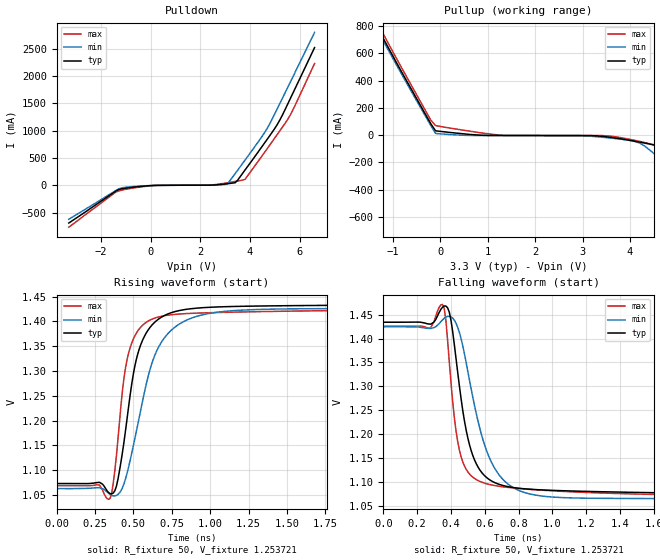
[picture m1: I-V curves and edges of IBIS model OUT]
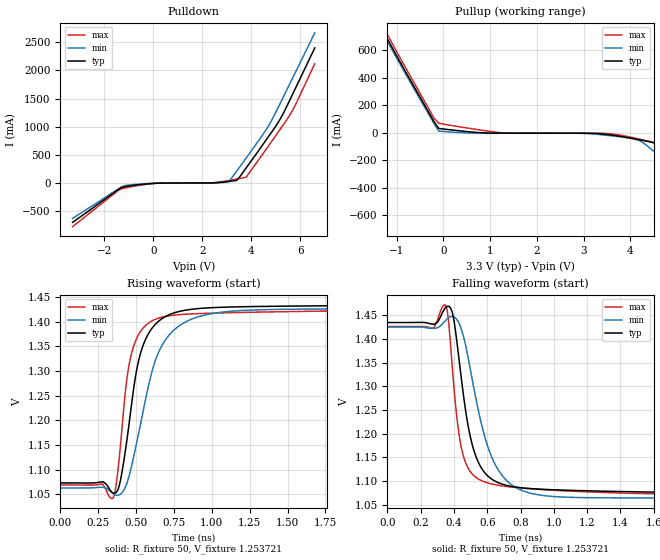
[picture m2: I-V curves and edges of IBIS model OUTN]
|   IBIS File of SG2520VHN C
|   LVDS, Vcc=3.3V, Io=3.5mA, fo>212.5MHz
[IBIS Ver]   3.2
[File Name]   sg2520vhn_hf_35m_33v.ibs
[File Rev]   1.0
[Date]   July 28, 2020
[Source]
Fairchild Ensigna Lab's Method
[Notes]
Created by Minoru Kozaki
[Disclaimer]
Seiko Epson Corporation makes no warranty with respect to the
information contained herein.
[Copyright]
Copyright(C) 2020, Seiko Epson Corporation. All rights reserved.
|   Component
[Component]   SG2520VHN
[Manufacturer]  Seiko Epson Corporation
[Package]
R_pkg   17.7m   NA   NA
L_pkg   235p   NA   NA
C_pkg   208f   NA   NA
[Pin]   signal_name   model_name   R_pin   L_pin   C_pin
1   OE/ST   NC
2   NC   NC
3   GND   GND
4   OUT   OUT   17.7m   235p   208f
5   OUTN   OUTN   10.4m   129p   221f
6   VCC   POWER
[Diff Pin] inv_pin  vdiff  tdelay_typ
4   5   0   0
| Models and submodels in the file (2): OUT (Output), OUTN (Output)
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|   Model OUT
[Model]   OUT
Model_type   Output
Polarity   Non-Inverting
Vref = 1.25
Vmeas = 1.25
Rref = 50
Cref = 0
C_comp   4.5p   4.5p   4.5p
[Temperature Range]   25   105   -40
[Voltage Range]   3.3   2.97   3.63
[Pullup Reference]   3.3   2.97   3.63
[Pulldown Reference]   0   0   0
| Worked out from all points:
|   slope of the pulldown table from 0 to 0.495 V, typ, clamps not added: 93.6 ohm
|   slope of the pullup table from 0 to 0.495 V, typ, clamps not added: 27.1 ohm
|   falling waveform, R_fixture 50, V_fixture 1.253721: 20-80 % time 111ps typ, 159ps min, 82ps max; typ from 1.43 V to 1.07 V
|   rising waveform, R_fixture 50, V_fixture 1.253721: 20-80 % time 126ps typ, 182ps min, 93.9ps max; typ from 1.07 V to 1.43 V
[Pullup]
-3.3V     2.52A      2.491A     2.553A
-1.4V     836.3mA    816.7mA    870.6mA
-1.3V     772mA      752.7mA    805.5mA
-1.2V     707.8mA    689.3mA    740.4mA
-200mV    82.37mA    68.93mA    109mA
-100mV    31.06mA    11.88mA    69.24mA
1.3V      -3.445mA   -3.542mA   -1.568mA
3.7V      -22.07mA   -26.28mA   -13.33mA
4.2V      -52.03mA   -58.34mA   -46.65mA
4.6V      -86.37mA   -162.6mA   -79.71mA
5.1V      -235.7mA   -303.2mA   -154.3mA
6.6V      -696.4mA   -716.3mA   -667mA
[Pulldown]
-3.3V     -688mA     -619.2mA   -763.3mA
-1.3V     -77.66mA   -65.14mA   -100.7mA
-900mV    -43.73mA   -28.15mA   -61.66mA
100mV     -787uA     -166.4uA   -2.717mA
2.3V      4.748mA    4.434mA    5.464mA
3.1V      32.02mA    32.24mA    48.87mA
3.4V      49.65mA    216.8mA    72.62mA
3.8V      283.6mA    464.3mA    111.6mA
4.6V      786.8mA    976.4mA    614.4mA
5.2V      1.197A     1.499A     999.8mA
5.7V      1.663A     1.963A     1.357A
6.6V      2.524A     2.802A     2.232A
[Falling Waveform]
R_fixture = 50
V_fixture = 1.253721
V_fixture_min = 1.243544
V_fixture_max = 1.247515
0s        1.434V     1.425V     1.426V
280ps     1.43V      1.421V     1.423V
350ps     1.466V     1.439V     1.471V
380ps     1.465V     1.446V     1.396V
420ps     1.387V     1.439V     1.234V
470ps     1.249V     1.384V     1.141V
560ps     1.131V     1.227V     1.102V
710ps     1.092V     1.104V     1.089V
1.1ns     1.081V     1.066V     1.079V
4ns       1.073V     1.063V     1.069V
[Rising Waveform]
R_fixture = 50
V_fixture = 1.253721
V_fixture_min = 1.243544
V_fixture_max = 1.247515
0s        1.073V     1.063V     1.069V
350ps     1.052V     1.051V     1.044V
400ps     1.082V     1.051V     1.162V
440ps     1.159V     1.073V     1.288V
470ps     1.23V      1.107V     1.337V
540ps     1.346V     1.209V     1.385V
660ps     1.404V     1.345V     1.409V
840ps     1.424V     1.402V     1.416V
1.15ns    1.43V      1.422V     1.419V
4ns       1.434V     1.425V     1.425V
[Ramp]
R_load = 50
dV/dt_r   0.21658/126.28p   0.21627/180.23p   0.21455/94.28p
dV/dt_f   0.21658/111.11p   0.21627/158.52p   0.21455/81.98p
|   Model OUTN
[Model]   OUTN
Model_type   Output
Polarity   Inverting
Vref = 1.250
Vmeas = 1.250
Rref = 50
Cref = 0
C_comp   4.5p   4.5p   4.5p
[Temperature Range]   25   105   -40
[Voltage Range]   3.3   2.97   3.63
[Pullup Reference]   3.3   2.97   3.63
[Pulldown Reference]   0   0   0
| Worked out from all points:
|   slope of the pulldown table from 0 to 0.495 V, typ, clamps not added: 93.5 ohm
|   slope of the pullup table from 0 to 0.495 V, typ, clamps not added: 27.2 ohm
|   falling waveform, R_fixture 50, V_fixture 1.253721: 20-80 % time 111ps typ, 158ps min, 81.8ps max; typ from 1.43 V to 1.07 V
|   rising waveform, R_fixture 50, V_fixture 1.253721: 20-80 % time 126ps typ, 182ps min, 94.2ps max; typ from 1.07 V to 1.43 V
[Pullup]
-3.3V     2.395A     2.371A     2.423A
-1.4V     807.3mA    788.2mA    840.5mA
-1.3V     745.2mA    726.6mA    777.6mA
-1.2V     683.3mA    665.4mA    714.8mA
-200mV    79.7mA     66.61mA    105.6mA
-100mV    31mA       11.87mA    69.04mA
1.3V      -3.445mA   -3.542mA   -1.57mA
3.7V      -22.11mA   -26.36mA   -13.35mA
4.2V      -52.16mA   -58.54mA   -46.8mA
4.6V      -86.46mA   -163.7mA   -80mA
5.1V      -236.9mA   -305.5mA   -153.8mA
6.6V      -702mA     -723mA     -671.6mA
[Pulldown]
-3.3V     -693.9mA   -625mA     -769mA
-1.3V     -77.82mA   -65.42mA   -100.8mA
-900mV    -43.8mA    -28.25mA   -61.8mA
100mV     -789.5uA   -167.7uA   -2.723mA
2.3V      4.748mA    4.435mA    5.466mA
3.1V      31.94mA    31.26mA    48.71mA
3.4V      49.52mA    209.4mA    72.36mA
3.8V      273.9mA    448.2mA    108.2mA
4.7V      821.2mA    1.009A     655.2mA
5.2V      1.147A     1.428A     965.6mA
5.7V      1.583A     1.87A      1.297A
6.6V      2.399A     2.666A     2.119A
[Falling Waveform]
R_fixture = 50
V_fixture = 1.253721
V_fixture_min = 1.243544
V_fixture_max = 1.247515
0s        1.434V     1.425V     1.426V
280ps     1.43V      1.422V     1.423V
350ps     1.466V     1.439V     1.471V
380ps     1.465V     1.447V     1.386V
420ps     1.388V     1.44V      1.227V
470ps     1.249V     1.387V     1.139V
560ps     1.131V     1.228V     1.102V
710ps     1.092V     1.104V     1.089V
1.1ns     1.081V     1.066V     1.079V
4ns       1.073V     1.063V     1.069V
[Rising Waveform]
R_fixture = 50
V_fixture = 1.253721
V_fixture_min = 1.243544
V_fixture_max = 1.247515
0s        1.073V     1.063V     1.069V
350ps     1.052V     1.051V     1.044V
400ps     1.084V     1.051V     1.161V
440ps     1.162V     1.073V     1.287V
470ps     1.233V     1.107V     1.336V
540ps     1.347V     1.209V     1.385V
660ps     1.404V     1.346V     1.408V
840ps     1.424V     1.402V     1.416V
1.15ns    1.43V      1.422V     1.419V
4ns       1.434V     1.425V     1.425V
[Ramp]
R_load = 50
dV/dt_r   0.21635/126.19p   0.21605/179.64p   0.21432/94.38p
dV/dt_f   0.21635/110.50p   0.21605/157.14p   0.21432/81.53p
